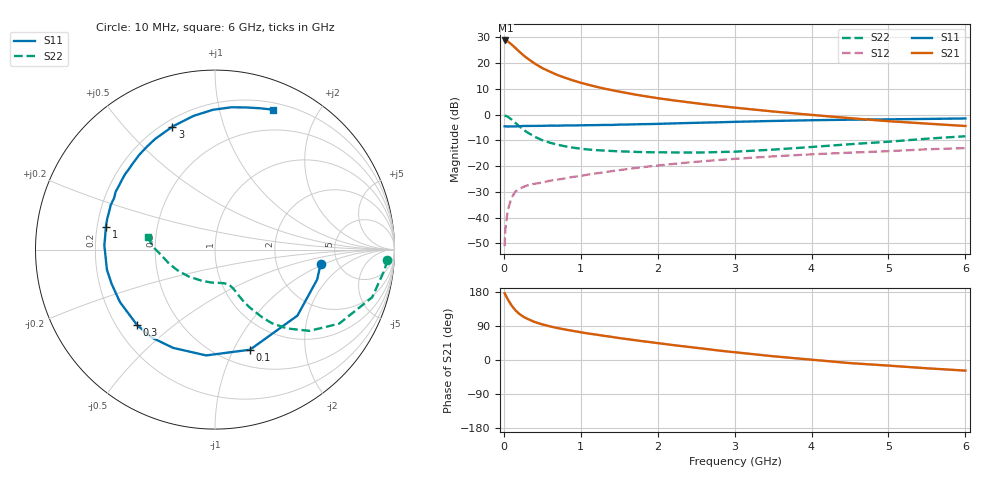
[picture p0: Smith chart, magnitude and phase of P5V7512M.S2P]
! SIEMENS Small Signal Semiconductors
! BFP183
! Si NPN RF Bipolar Junction Transistor in SOT143
! VCE = 0.75 V  IC = 12 mA
! Common Emitter S-Parameters:  March  1996
# GHz  S  MA  R  50
!  f  S11  S21  S12  S22
! GHz  MAG  ANG  MAG  ANG  MAG  ANG  MAG  ANG
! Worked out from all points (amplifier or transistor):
!   36 points, 10 MHz to 6 GHz, reference 50 ohm
!   highest |S21| = 28.8 dB at 20 MHz (marker M1)
!   |S21| within 3 dB of that: start of sweep to 153.2 MHz
!   unconditionally stable (mu >= 1): 847.6 MHz to end of sweep
!   at 250 MHz: K = 0.41, MSG = 25.6 dB, |S12| = -28.1 dB
!   at 1.4 GHz: K = 1.21, MAG = 13.0 dB, |S12| = -21.9 dB
!   at 6 GHz: K = 1.06, MAG = 2.8 dB, |S12| = -13.0 dB
!   S11 on the Smith chart (normalised r, x): 10 MHz: 3.68, -0.92; 100 MHz: 0.68, -1.16; 300 MHz: 0.28, -0.38; 1 GHz: 0.24, +0.10; 3 GHz: 0.24, +0.69; 6 GHz: 0.27, +1.46
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0.01  0.5938 -7.8  27.54 176.2  0.0028 85.1  0.9618 -3.4
0.02  0.5931 -16.3  27.56 172.4  0.006 78.7  0.9511 -6.9
0.05  0.5884 -38.7  26.51 160.4  0.0137 75.8  0.9151 -16.9
0.1  0.5909 -70.7  23.07 144.1  0.0244 60.7  0.8056 -30.8
0.15  0.5917 -94.8  19.71 131.2  0.032 52.5  0.6944 -40.7
0.2  0.5952 -113.1  16.8 121.8  0.0362 46.4  0.5949 -47.6
0.25  0.6036 -125.7  14.38 114.7  0.0392 43.2  0.5184 -52.3
0.3  0.6042 -135.9  12.55 109.2  0.0422 41.5  0.4583 -55.2
0.4  0.605 -151.0  9.846 100.3  0.0455 39.5  0.3732 -59.2
0.5  0.6068 -161.6  8.012 94.0  0.0482 38.1  0.3198 -61.5
0.6  0.6126 -169.4  6.831 88.7  0.0522 39.2  0.2851 -62.8
0.7  0.6109 -176.2  5.851 84.3  0.0549 40.0  0.2602 -63.8
0.8  0.6171 177.9  5.179 80.3  0.0581 40.7  0.2425 -64.8
1  0.6212 168.1  4.157 73.2  0.0647 42.1  0.2182 -67.1
1.1  0.6246 164.1  3.802 69.8  0.0689 42.5  0.2105 -68.5
1.5  0.6406 149.8  2.798 57.9  0.0837 43.1  0.194 -75.0
2.2  0.6759 128.7  1.898 39.4  0.1106 40.6  0.1846 -92.5
3  0.7253 109.1  1.369 20.5  0.1388 34.9  0.1909 -118.0
3.5  0.7546 99.1  1.152 9.9  0.1549 30.9  0.2095 -134.4
4.5  0.7983 83.4  0.855 -8.2  0.183 22.3  0.267 -162.7
5.5  0.8265 72.3  0.67 -21.9  0.2127 14.7  0.3414 178.1
6  0.8437 67.6  0.602 -28.0  0.2243 10.1  0.3811 169.8
